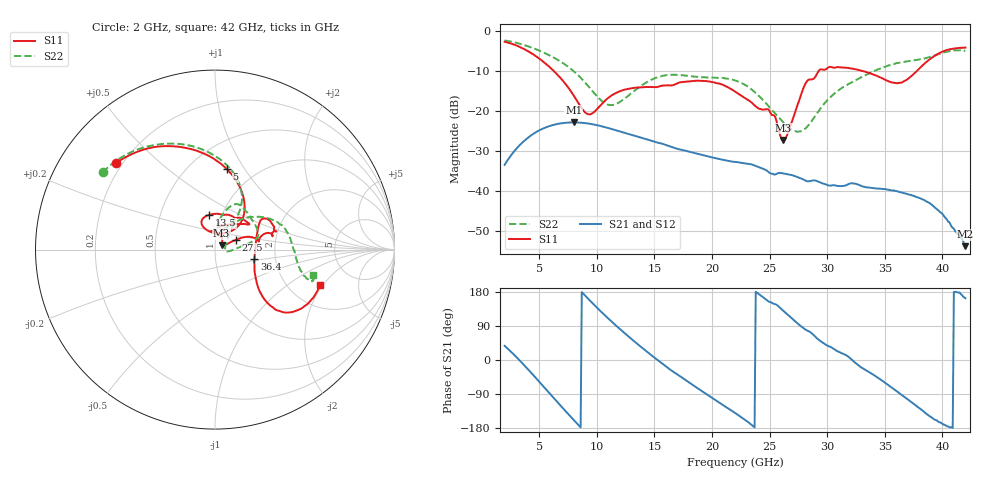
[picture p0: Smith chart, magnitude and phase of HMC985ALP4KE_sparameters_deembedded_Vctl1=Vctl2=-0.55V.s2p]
!s2p File: Measurements: S11, S21, S12, S22
# GHz S dB R 50.0
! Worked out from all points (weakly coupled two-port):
!   401 points, 2 GHz to 42 GHz, reference 50 ohm
!   highest |S21| = -22.82 dB at 8 GHz (marker M1); lowest = -53.7 dB at 42 GHz (marker M2)
!   lowest |S11| = -27.2 dB at 26.2 GHz (marker M3), VSWR 1.09, Z = 53.7 + j2.55 ohm
!   |S11| at or under -10 dB: 6.27 GHz to 29.26 GHz (22.99 GHz wide, 129 % of centre); 33.1 GHz to 37.79 GHz (4.686 GHz wide, 13.2 % of centre)
!   |S22| runs from -25.2 to -2.4 dB; largest |S21 - S12| = 0.00015
!   S11 on the Smith chart (normalised r, x): 2 GHz: 0.18, +0.36; 5 GHz: 0.74, +0.84; 13.5 GHz: 0.87, +0.35; 27.5 GHz: 1.25, +0.14; 36.4 GHz: 1.55, -0.17; 42 GHz: 2.95, -1.88
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2  -2.71 139.0  -33.42 37.5  -33.43 37.5  -2.39 145.4
3.4  -4.12 112.3  -28.24 -4.2  -28.24 -4.2  -3.28 123.0
5  -6.89 81.5  -24.82 -57.1  -24.82 -57.1  -4.90 98.4
8  -16.13 46.5  -22.82 -158.3  -22.83 -158.3  -10.06 61.4
8.7  -19.33 58.2  -22.91 179.1  -22.92 179.1  -11.99 57.4
9.5  -20.74 89.9  -23.21 154.0  -23.22 154.0  -14.57 56.6
11.1  -16.48 117.8  -24.30 106.6  -24.31 106.6  -18.49 72.6
13.5  -14.13 100.0  -26.32 43.1  -26.33 43.1  -14.42 78.9
15.4  -13.88 73.9  -27.94 -2.6  -27.94 -2.6  -11.44 68.3
18.9  -12.46 37.4  -30.78 -77.4  -30.78 -77.4  -11.50 40.5
22  -15.11 53.8  -32.67 -139.5  -32.69 -139.5  -12.36 15.1
24.9  -19.59 96.1  -35.16 154.7  -35.16 154.7  -18.71 2.4
26.2  -27.22 33.0  -35.54 129.6  -35.55 129.5  -22.83 -8.2
27.5  -17.90 24.9  -36.54 94.7  -36.54 94.7  -25.11 1.9
28.1  -13.23 18.5  -37.29 80.5  -37.34 80.4  -24.37 18.5
28.7  -12.08 11.1  -37.33 69.4  -37.35 69.5  -22.30 33.1
31  -9.05 21.7  -38.70 21.7  -38.71 21.8  -14.77 52.7
33.3  -10.18 33.0  -38.97 -25.4  -38.98 -25.5  -11.09 40.7
35.4  -12.63 11.5  -39.64 -68.3  -39.64 -68.5  -8.59 25.1
36.4  -12.93 -13.7  -40.26 -90.4  -40.23 -90.8  -7.82 16.8
39.5  -5.95 -43.2  -44.38 -159.0  -44.37 -159.5  -5.93 -14.9
42  -4.16 -18.5  -53.69 162.9  -53.98 162.6  -4.95 -14.3
